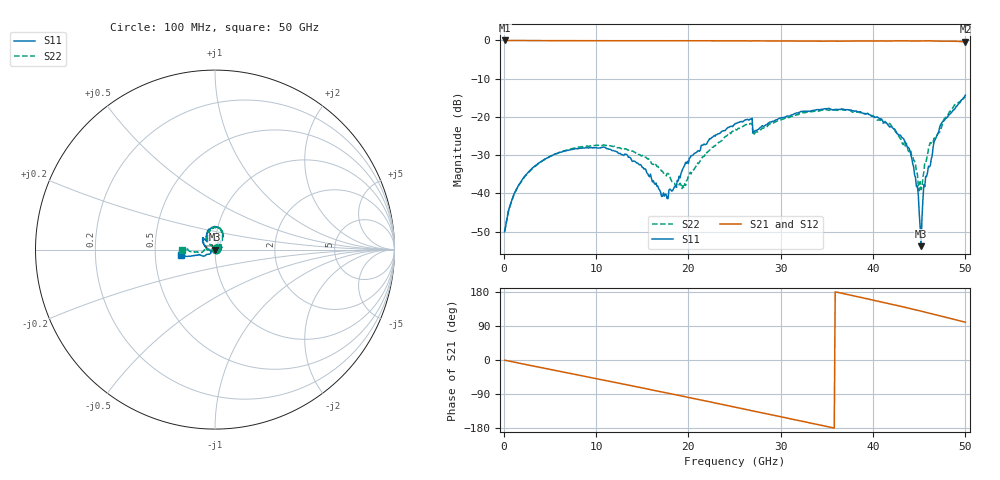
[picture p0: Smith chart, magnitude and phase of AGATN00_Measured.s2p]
! Filename4Jim: AG16_W2_AGATN00_E_1505_LRM_1BW_LRM.s2p
! Calibration: AG02 LRM + TRL
! Notes:
! Row:15, Col:5
! Probes: nan
! Prober: MPI TS150
! Date: 2023-09-21 11:09:00
! DC: None
# GHz S dB R 50
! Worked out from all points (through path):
!   500 points, 100 MHz to 50 GHz, reference 50 ohm
!   highest |S21| = -0.03 dB at 100 MHz (marker M1); lowest = -0.4 dB at 50 GHz (marker M2)
!   group delay of S21, straight-line fit = 14.3 ps
!   lowest |S11| = -53.8 dB at 45.2 GHz (marker M3), VSWR 1.00, Z = 49.8 - j0.1 ohm
!   |S11| at or under -10 dB: start of sweep to end of sweep
!   |S22| runs from -50.0 to -14.7 dB; largest |S21 - S12| = 0.0032
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0.1  -50.00 22.0  -0.03 -0.5  -0.02 -0.5  -49.96 23.0
1.1  -40.30 56.4  -0.04 -5.5  -0.04 -5.5  -40.41 57.9
2.7  -34.36 58.5  -0.05 -13.4  -0.05 -13.4  -34.51 61.4
8.5  -28.17 34.3  -0.09 -41.8  -0.09 -41.8  -27.76 46.6
13.3  -29.79 3.3  -0.10 -65.3  -0.10 -65.3  -28.47 32.8
16.8  -38.87 -58.8  -0.10 -82.7  -0.09 -82.8  -33.37 36.1
17.6  -40.33 -100.7  -0.11 -86.7  -0.11 -86.7  -35.40 47.2
19.5  -33.06 -157.8  -0.10 -96.1  -0.09 -96.2  -38.63 102.2
21.7  -27.09 170.4  -0.11 -107.2  -0.10 -107.3  -30.35 132.6
25.1  -21.72 147.2  -0.11 -124.5  -0.11 -124.6  -23.26 127.6
26.7  -20.54 135.2  -0.14 -132.7  -0.14 -132.7  -21.70 121.4
27.2  -23.64 133.3  -0.13 -135.4  -0.13 -135.4  -24.17 126.9
33.4  -18.37 100.8  -0.19 -167.2  -0.19 -167.3  -18.64 97.8
38.4  -18.65 74.9  -0.20 166.7  -0.19 166.6  -18.70 74.5
41.7  -22.30 57.3  -0.18 148.9  -0.17 148.8  -21.92 62.3
44  -28.84 44.9  -0.16 135.8  -0.16 135.7  -28.66 68.7
44.7  -38.21 46.2  -0.16 132.0  -0.16 131.8  -34.32 77.4
45  -45.16 26.6  -0.15 130.1  -0.14 130.1  -39.30 107.7
45.2  -53.78 -150.5  -0.15 129.0  -0.15 128.9  -39.00 138.1
45.7  -35.52 -161.4  -0.14 126.2  -0.14 126.0  -32.05 174.0
46.8  -25.53 -149.6  -0.20 119.4  -0.20 119.3  -25.34 -179.8
50  -14.31 -170.2  -0.36 99.7  -0.35 99.5  -14.70 -179.4
